(* Logix 5000 AddOnInstructionDefinition export Banner_DXMR_IOLM_Param_v5; software revision 33.00 *)

TYPE Banner_IOL_Port_v5 :   // UDT that has all of the data items necessary to communicate with a specific Port on a IO-Link Master
STRUCT
   Port_Controlled : INT;   // Each bit represents a port on an IO-Link Master. Set to 1 to tell AOI to control that port.
   Port_Activate : INT;   // Each bit represents a port on an IO-Link Master. When ON that port will process any commands in queue.
   Port_Read : INT;   // Each bit represents a port on an IO-Link Master. Used to determine when device AOI has requested a Read command.
   Port_Write : INT;   // Each bit represents a port on an IO-Link Master. Used to determine when device AOI has requested a Write command.
   Port_RW_Complete : INT;   // Each bit represents a port on an IO-Link Master. Tells device AOI that Read or Write request has been completed.
   Port_Device_Read : INT;
   Data_Transfer : SINT[250];   // Array to transfer data from IO-Master to device AOIs.
END_STRUCT
END_TYPE

TYPE Banner_IOLM_EL_v5 :   // Error Log for Messages to IOLM.
STRUCT
   RW : SINT;   // 0 = Read, 1 = Write.
   Port : SINT;   // Port number that generated error.
   Index : INT;   // IO-Link Index for generated error.
END_STRUCT
END_TYPE

TYPE Banner_IOLM_v5 :   // UDT to control IO-Link Masters.
STRUCT
   Message_Source_Data : SINT[260];
   Message_Destination_Data : SINT[260];
   Error_Log : Banner_IOLM_EL_v5[10];
   Error_Write_Retry : BOOL;
   Num_Error_MSGS : DINT;
   IO_Link_Master_Busy : BOOL;   // 0 = While waiting for a command, 1 = Processing command
   AOI_Reset : BOOL;
   Port_Data : Banner_IOL_Port_v5;   // All of the necessary data to work with the various ports of the IO-Link Master.
   Halt_Operation : BOOL;   // When parameter is 1 the AOI is halted as next available time frame.
   AOI_Halted : BOOL;   // AOI is in standby mode until Halt Operation tag is set back to 0.
END_STRUCT
END_TYPE

ADD_ON_INSTRUCTION Banner_DXMR_IOLM_Param_v5   (* revision 5.0, vendor Banner Engineering *)
// AOI that controls a Banner IO-Link Master with IO-Link Devices
// Revision note:
// Added Port Control functionality. This should simplify the setup. Also added links for direct connection to the Input and Output Assmebly Instances.
VAR_IN_OUT
   IOLM : Banner_IOLM_v5; {required}
   Input : SINT[456]; {required}
   Output : SINT[456]; {required}
END_VAR
VAR_INPUT
   Port1 : BOOL; {required}
   Port2 : BOOL; {required}
   Port3 : BOOL; {required}
   Port4 : BOOL; {required}
   Port5 : BOOL; {required}
   Port6 : BOOL; {required}
   Port7 : BOOL; {required}
   Port8 : BOOL; {required}
END_VAR
VAR_OUTPUT
   Done : BOOL; {visible}
   Busy : BOOL; {visible}
   Error : BOOL; {visible}
END_VAR
VAR
   Lock : DINT; {access None}
   Byte_Length : SINT; {access None}
   Current_Port : INT; {access None}   // Current port to communicate with via the IO-Link Master.
   Timer : TIMER := (PRE := 500); {access None}
   Error_Index : DINT; {access None}
   Timer2 : TIMER := (PRE := 5000); {access None}
   Temp_Index : INT; {access None}
   ErrCount : DINT; {access None}
   Timer4 : TIMER := (PRE := 2000); {access None}
   Timer5 : TIMER := (PRE := 2000); {access None}
   Timer3 : TIMER := (PRE := 2000); {access None}
   Timer6 : TIMER := (PRE := 3000); {access None}
   Timer7 : TIMER := (PRE := 3000); {access None}
   Timer8 : TIMER := (PRE := 3000); {access None}
   Write_Index : DINT; {access None}
   WriteTimer : TIMER := (PRE := 60000); {access None}
   WriteCnt : DINT; {access None}
   Last_Index : DINT; {access None}
   WrCntTotal : DINT; {access None}
END_VAR

ROUTINE Logic   (* ladder *)
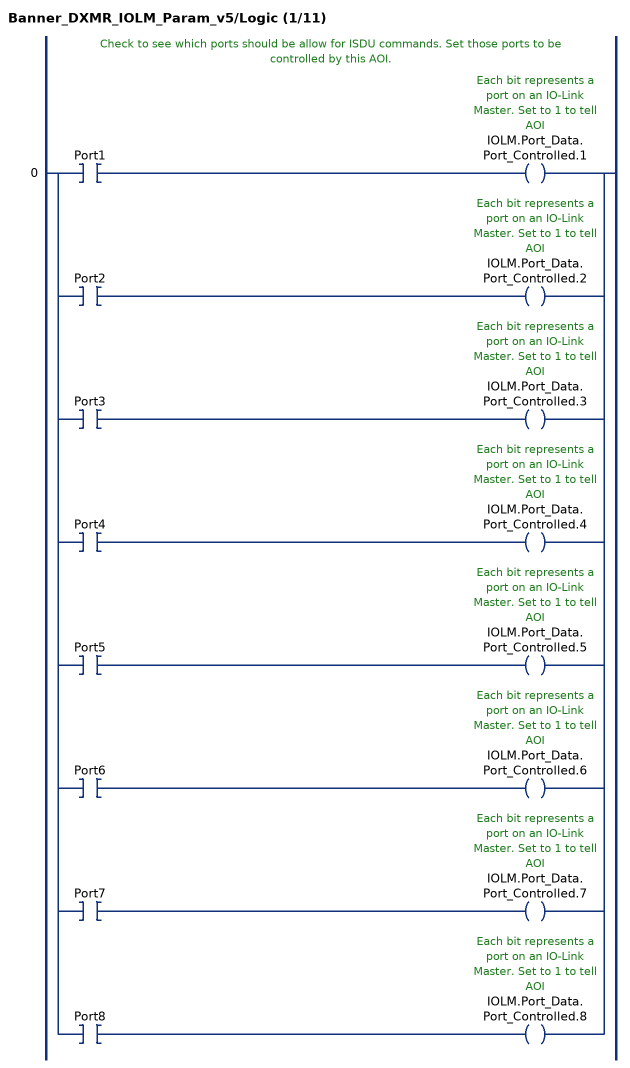
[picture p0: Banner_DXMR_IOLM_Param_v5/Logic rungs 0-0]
   // Check to see which ports should be allow for ISDU commands. Set those ports to be controlled by this AOI.
   0: [XIC(Port1) OTE(IOLM.Port_Data.Port_Controlled.1) ,XIC(Port2) OTE(IOLM.Port_Data.Port_Controlled.2) ,XIC(Port3) OTE(IOLM.Port_Data.Port_Controlled.3) ,XIC(Port4) OTE(IOLM.Port_Data.Port_Controlled.4) ,XIC(Port5) OTE(IOLM.Port_Data.Port_Controlled.5) ,XIC(Port6) OTE(IOLM.Port_Data.Port_Controlled.6) ,XIC(Port7) OTE(IOLM.Port_Data.Port_Controlled.7) ,XIC(Port8) OTE(IOLM.Port_Data.Port_Controlled.8) ];
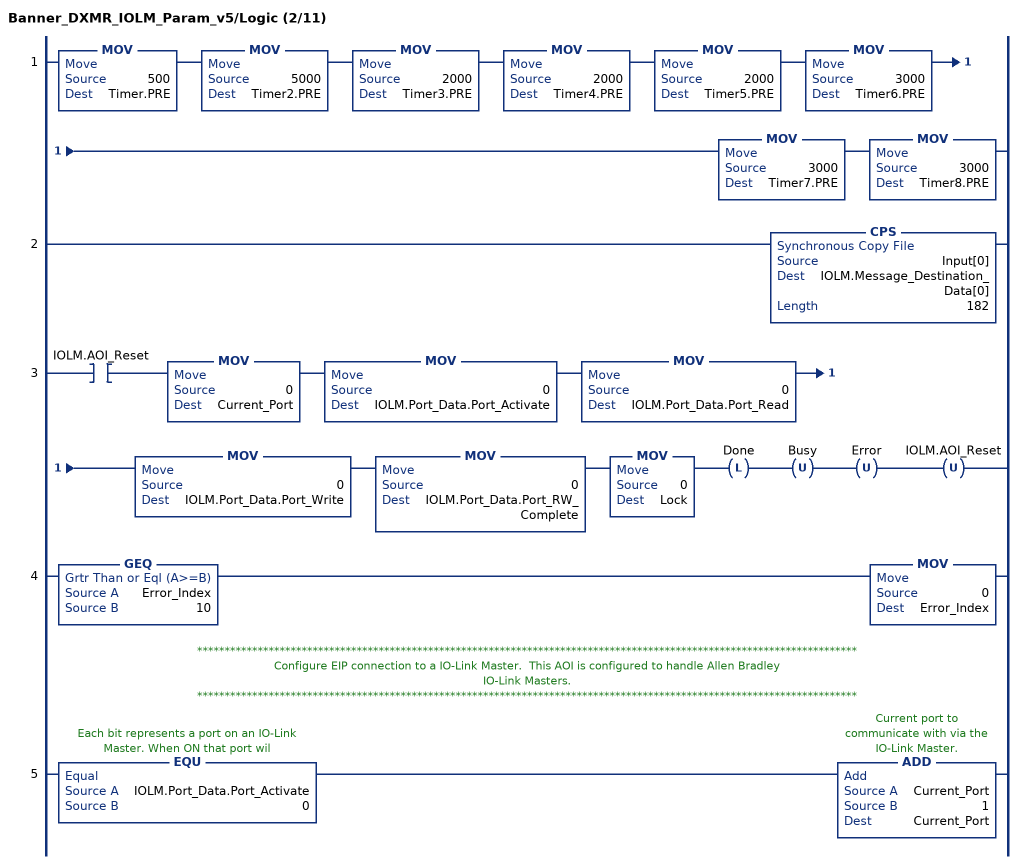
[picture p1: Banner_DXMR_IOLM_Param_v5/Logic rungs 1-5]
   1: MOV(500,Timer.PRE)MOV(5000,Timer2.PRE)MOV(2000,Timer3.PRE)MOV(2000,Timer4.PRE)MOV(2000,Timer5.PRE)MOV(3000,Timer6.PRE)MOV(3000,Timer7.PRE)MOV(3000,Timer8.PRE);
   2: CPS(Input[0],IOLM.Message_Destination_Data[0],182);
   3: XIC(IOLM.AOI_Reset)MOV(0,Current_Port)MOV(0,IOLM.Port_Data.Port_Activate)MOV(0,IOLM.Port_Data.Port_Read)MOV(0,IOLM.Port_Data.Port_Write)MOV(0,IOLM.Port_Data.Port_RW_Complete)MOV(0,Lock)OTL(Done)OTU(Busy)OTU(Error)OTU(IOLM.AOI_Reset);
   4: GEQ(Error_Index,10)MOV(0,Error_Index);
   // ************************************************************************************************************************
   // Configure EIP connection to a IO-Link Master.  This AOI is configured to handle Allen Bradley
   // IO-Link Masters.
   // ************************************************************************************************************************
   5: EQU(IOLM.Port_Data.Port_Activate,0)ADD(Current_Port,1,Current_Port);
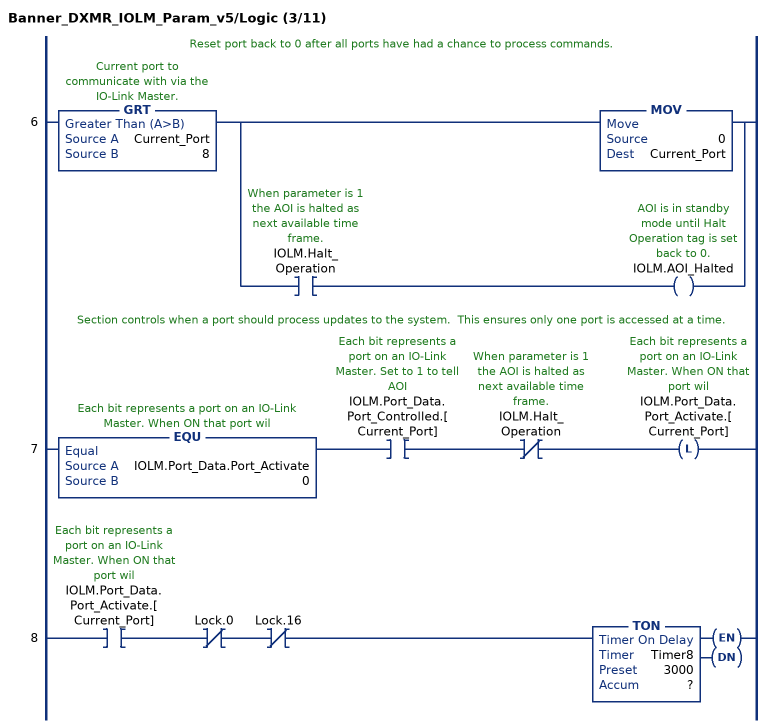
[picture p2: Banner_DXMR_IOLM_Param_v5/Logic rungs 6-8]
   // Reset port back to 0 after all ports have had a chance to process commands.
   6: GRT(Current_Port,8)[MOV(0,Current_Port) ,XIC(IOLM.Halt_Operation) OTE(IOLM.AOI_Halted) ];
   // Section controls when a port should process updates to the system.  This ensures only one port is accessed at a time.
   7: EQU(IOLM.Port_Data.Port_Activate,0)XIC(IOLM.Port_Data.Port_Controlled.[Current_Port])XIO(IOLM.Halt_Operation)OTL(IOLM.Port_Data.Port_Activate.[Current_Port]);
   8: XIC(IOLM.Port_Data.Port_Activate.[Current_Port])XIO(Lock.0)XIO(Lock.16)TON(Timer8,?,?);
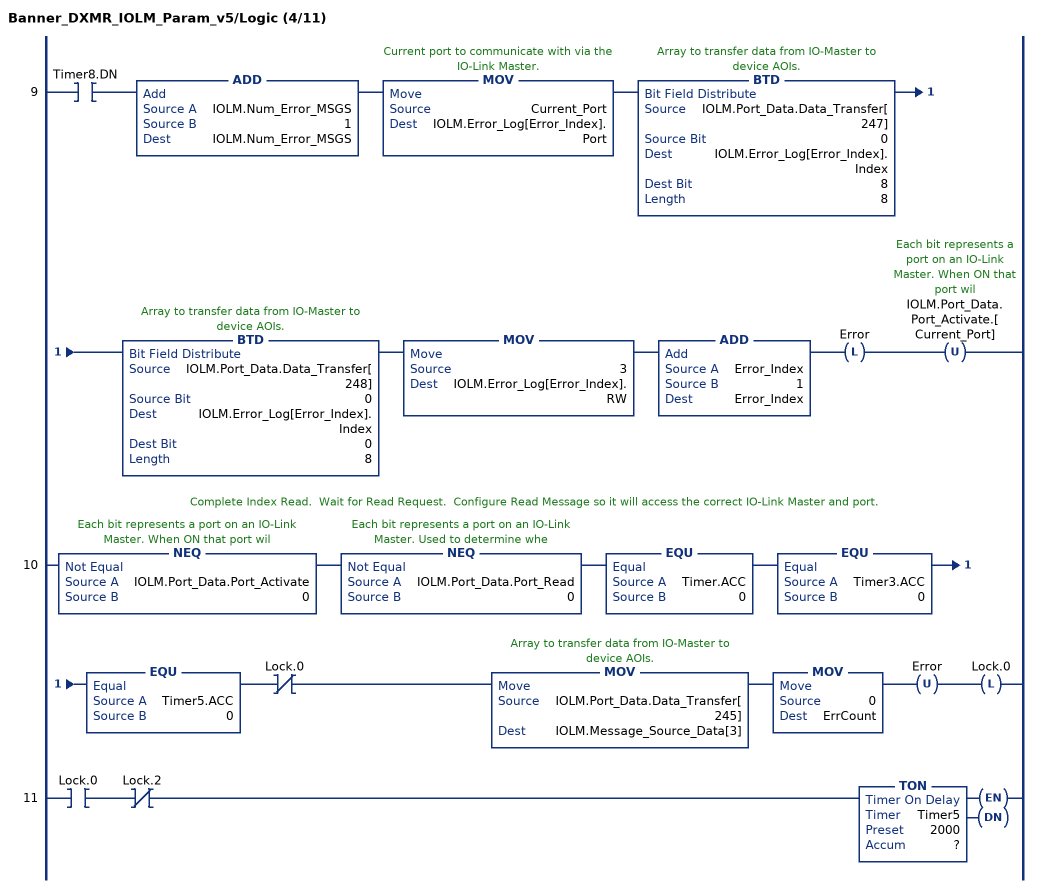
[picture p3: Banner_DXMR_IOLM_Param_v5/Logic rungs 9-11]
   9: XIC(Timer8.DN)ADD(IOLM.Num_Error_MSGS,1,IOLM.Num_Error_MSGS)MOV(Current_Port,IOLM.Error_Log[Error_Index].Port)BTD(IOLM.Port_Data.Data_Transfer[247],0,IOLM.Error_Log[Error_Index].Index,8,8)BTD(IOLM.Port_Data.Data_Transfer[248],0,IOLM.Error_Log[Error_Index].Index,0,8)MOV(3,IOLM.Error_Log[Error_Index].RW)ADD(Error_Index,1,Error_Index)OTL(Error)OTU(IOLM.Port_Data.Port_Activate.[Current_Port]);
   // Complete Index Read.  Wait for Read Request.  Configure Read Message so it will access the correct IO-Link Master and port.
   10: NEQ(IOLM.Port_Data.Port_Activate,0)NEQ(IOLM.Port_Data.Port_Read,0)EQU(Timer.ACC,0)EQU(Timer3.ACC,0)EQU(Timer5.ACC,0)XIO(Lock.0)MOV(IOLM.Port_Data.Data_Transfer[245],IOLM.Message_Source_Data[3])MOV(0,ErrCount)OTU(Error)OTL(Lock.0);
   11: XIC(Lock.0)XIO(Lock.2)TON(Timer5,?,?);
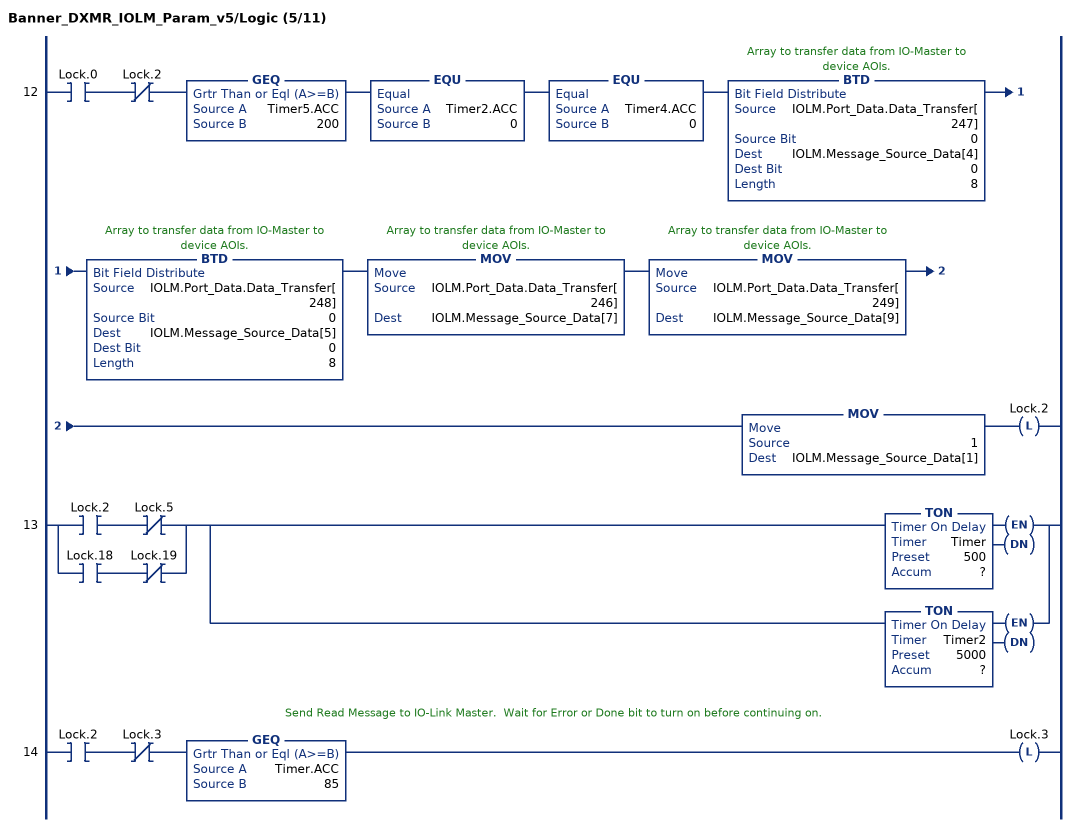
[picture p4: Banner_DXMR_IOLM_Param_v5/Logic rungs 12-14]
   12: XIC(Lock.0)XIO(Lock.2)GEQ(Timer5.ACC,200)EQU(Timer2.ACC,0)EQU(Timer4.ACC,0)BTD(IOLM.Port_Data.Data_Transfer[247],0,IOLM.Message_Source_Data[4],0,8)BTD(IOLM.Port_Data.Data_Transfer[248],0,IOLM.Message_Source_Data[5],0,8)MOV(IOLM.Port_Data.Data_Transfer[246],IOLM.Message_Source_Data[7])MOV(IOLM.Port_Data.Data_Transfer[249],IOLM.Message_Source_Data[9])MOV(1,IOLM.Message_Source_Data[1])OTL(Lock.2);
   13: [XIC(Lock.2) XIO(Lock.5) ,XIC(Lock.18) XIO(Lock.19) ][TON(Timer,?,?) ,TON(Timer2,?,?) ];
   // Send Read Message to IO-Link Master.  Wait for Error or Done bit to turn on before continuing on.
   14: XIC(Lock.2)XIO(Lock.3)GEQ(Timer.ACC,85)OTL(Lock.3);
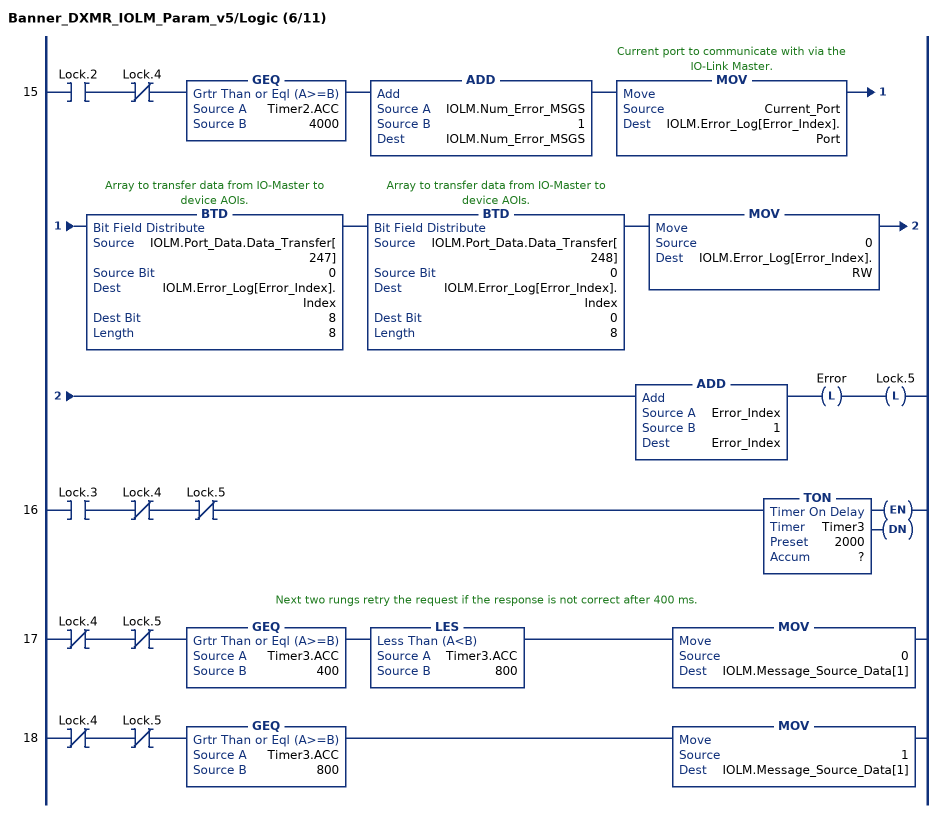
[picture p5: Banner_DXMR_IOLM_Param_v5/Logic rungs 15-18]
   15: XIC(Lock.2)XIO(Lock.4)GEQ(Timer2.ACC,4000)ADD(IOLM.Num_Error_MSGS,1,IOLM.Num_Error_MSGS)MOV(Current_Port,IOLM.Error_Log[Error_Index].Port)BTD(IOLM.Port_Data.Data_Transfer[247],0,IOLM.Error_Log[Error_Index].Index,8,8)BTD(IOLM.Port_Data.Data_Transfer[248],0,IOLM.Error_Log[Error_Index].Index,0,8)MOV(0,IOLM.Error_Log[Error_Index].RW)ADD(Error_Index,1,Error_Index)OTL(Error)OTL(Lock.5);
   16: XIC(Lock.3)XIO(Lock.4)XIO(Lock.5)TON(Timer3,?,?);
   // Next two rungs retry the request if the response is not correct after 400 ms.
   17: XIO(Lock.4)XIO(Lock.5)GEQ(Timer3.ACC,400)LES(Timer3.ACC,800)MOV(0,IOLM.Message_Source_Data[1]);
   18: XIO(Lock.4)XIO(Lock.5)GEQ(Timer3.ACC,800)MOV(1,IOLM.Message_Source_Data[1]);
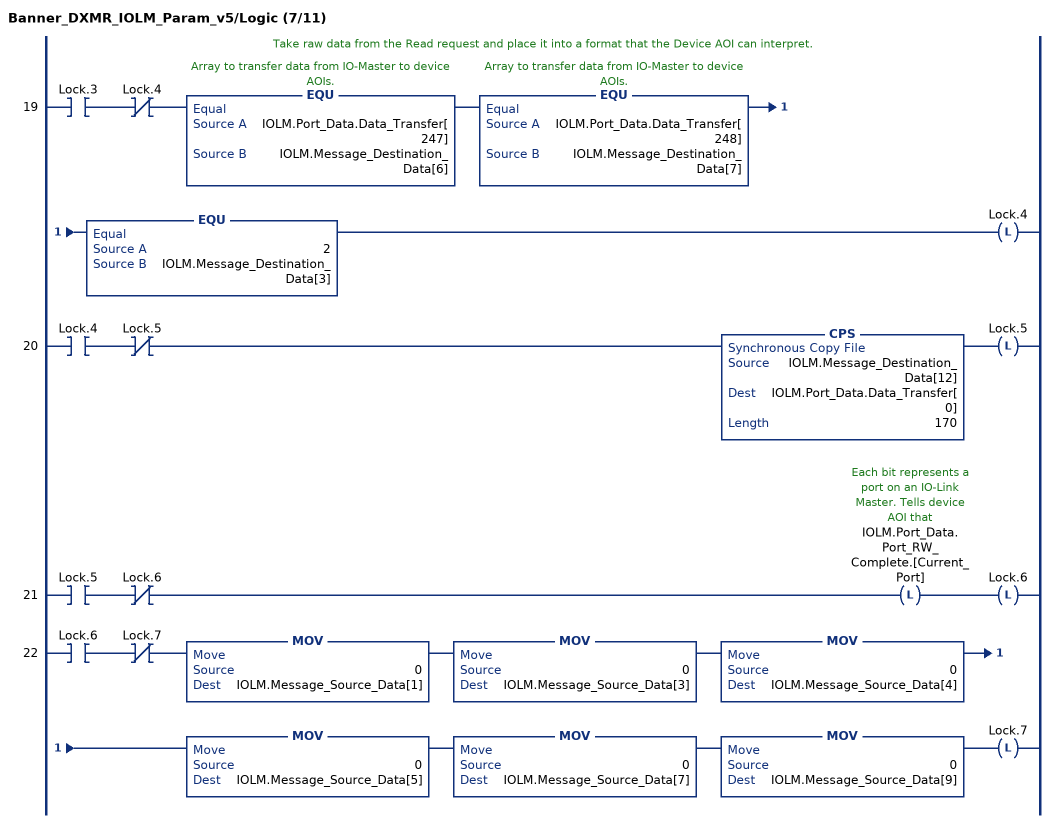
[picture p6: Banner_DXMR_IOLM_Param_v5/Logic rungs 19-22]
   // Take raw data from the Read request and place it into a format that the Device AOI can interpret.
   19: XIC(Lock.3)XIO(Lock.4)EQU(IOLM.Port_Data.Data_Transfer[247],IOLM.Message_Destination_Data[6])EQU(IOLM.Port_Data.Data_Transfer[248],IOLM.Message_Destination_Data[7])EQU(2,IOLM.Message_Destination_Data[3])OTL(Lock.4);
   20: XIC(Lock.4)XIO(Lock.5)CPS(IOLM.Message_Destination_Data[12],IOLM.Port_Data.Data_Transfer[0],170)OTL(Lock.5);
   21: XIC(Lock.5)XIO(Lock.6)OTL(IOLM.Port_Data.Port_RW_Complete.[Current_Port])OTL(Lock.6);
   22: XIC(Lock.6)XIO(Lock.7)MOV(0,IOLM.Message_Source_Data[1])MOV(0,IOLM.Message_Source_Data[3])MOV(0,IOLM.Message_Source_Data[4])MOV(0,IOLM.Message_Source_Data[5])MOV(0,IOLM.Message_Source_Data[7])MOV(0,IOLM.Message_Source_Data[9])OTL(Lock.7);
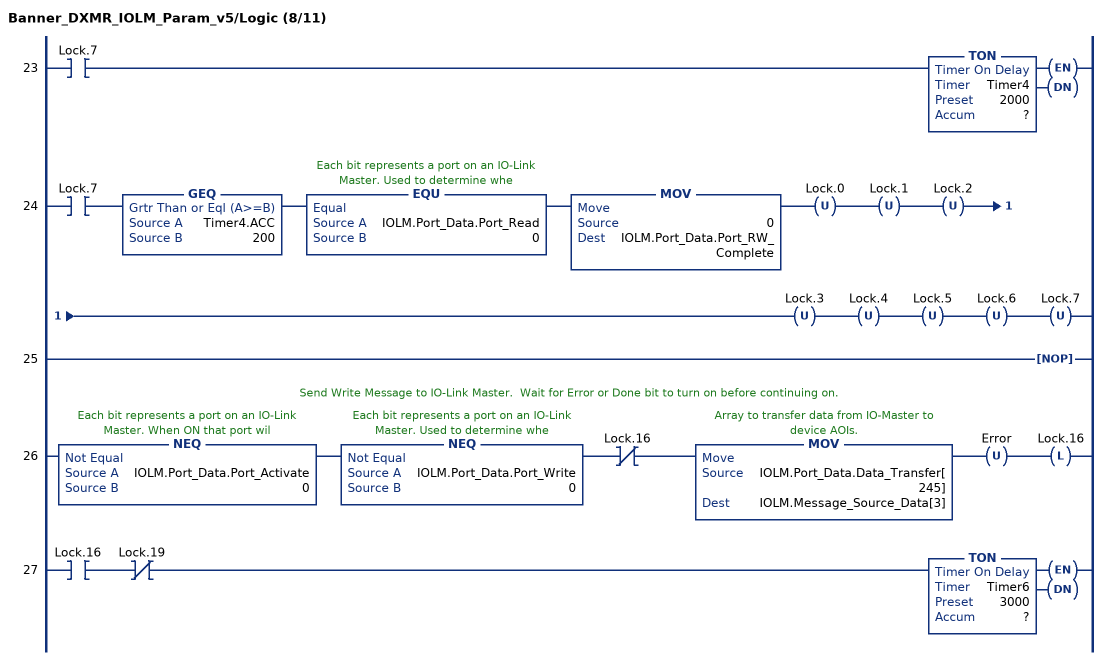
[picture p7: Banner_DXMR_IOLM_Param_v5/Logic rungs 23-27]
   23: XIC(Lock.7)TON(Timer4,?,?);
   24: XIC(Lock.7)GEQ(Timer4.ACC,200)EQU(IOLM.Port_Data.Port_Read,0)MOV(0,IOLM.Port_Data.Port_RW_Complete)OTU(Lock.0)OTU(Lock.1)OTU(Lock.2)OTU(Lock.3)OTU(Lock.4)OTU(Lock.5)OTU(Lock.6)OTU(Lock.7);
   25: NOP();
   // Send Write Message to IO-Link Master.  Wait for Error or Done bit to turn on before continuing on.
   26: NEQ(IOLM.Port_Data.Port_Activate,0)NEQ(IOLM.Port_Data.Port_Write,0)XIO(Lock.16)MOV(IOLM.Port_Data.Data_Transfer[245],IOLM.Message_Source_Data[3])OTU(Error)OTL(Lock.16);
   27: XIC(Lock.16)XIO(Lock.19)TON(Timer6,?,?);
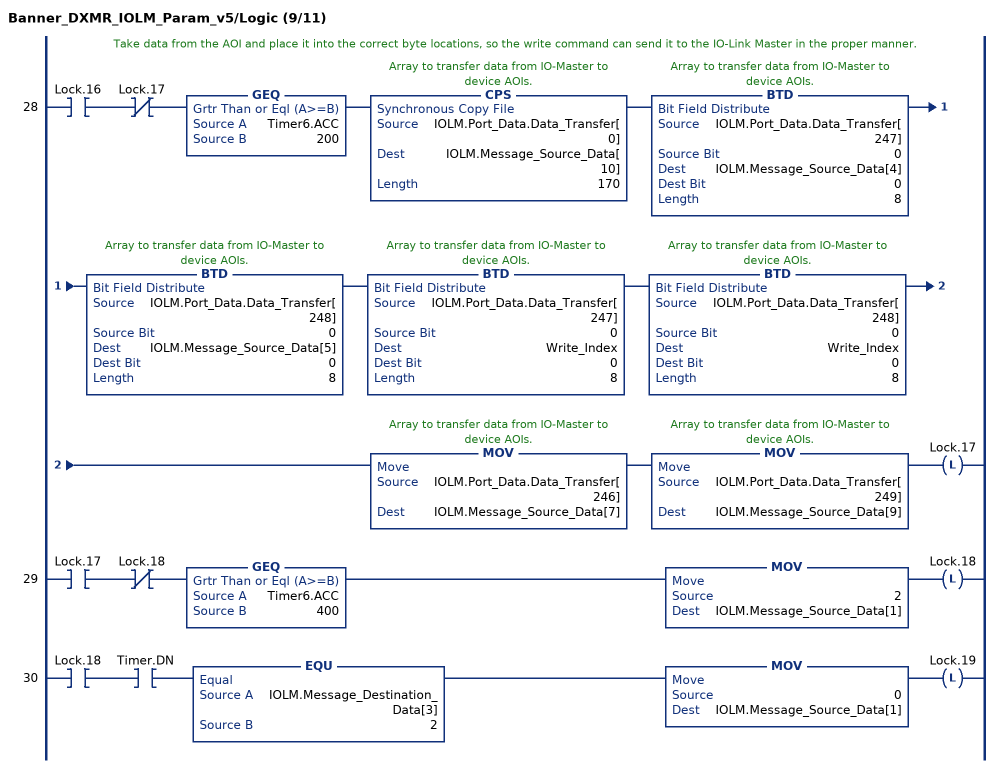
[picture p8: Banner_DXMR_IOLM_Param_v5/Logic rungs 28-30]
   // Take data from the AOI and place it into the correct byte locations, so the write command can send it to the IO-Link Master in the proper manner.
   28: XIC(Lock.16)XIO(Lock.17)GEQ(Timer6.ACC,200)CPS(IOLM.Port_Data.Data_Transfer[0],IOLM.Message_Source_Data[10],170)BTD(IOLM.Port_Data.Data_Transfer[247],0,IOLM.Message_Source_Data[4],0,8)BTD(IOLM.Port_Data.Data_Transfer[248],0,IOLM.Message_Source_Data[5],0,8)BTD(IOLM.Port_Data.Data_Transfer[247],0,Write_Index,0,8)BTD(IOLM.Port_Data.Data_Transfer[248],0,Write_Index,0,8)MOV(IOLM.Port_Data.Data_Transfer[246],IOLM.Message_Source_Data[7])MOV(IOLM.Port_Data.Data_Transfer[249],IOLM.Message_Source_Data[9])OTL(Lock.17);
   29: XIC(Lock.17)XIO(Lock.18)GEQ(Timer6.ACC,400)MOV(2,IOLM.Message_Source_Data[1])OTL(Lock.18);
   30: XIC(Lock.18)XIC(Timer.DN)EQU(IOLM.Message_Destination_Data[3],2)MOV(0,IOLM.Message_Source_Data[1])OTL(Lock.19);
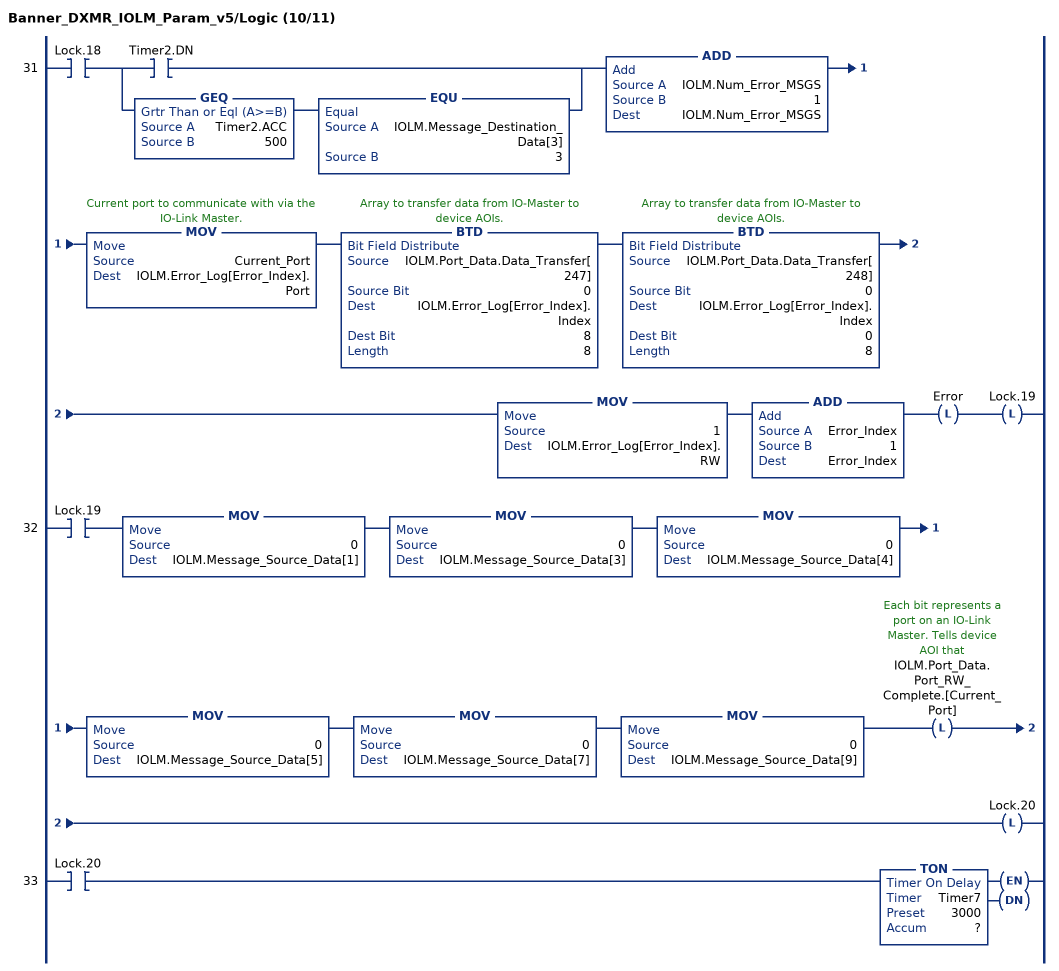
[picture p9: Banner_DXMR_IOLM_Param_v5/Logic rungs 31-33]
   31: XIC(Lock.18)[XIC(Timer2.DN) ,GEQ(Timer2.ACC,500) EQU(IOLM.Message_Destination_Data[3],3) ]ADD(IOLM.Num_Error_MSGS,1,IOLM.Num_Error_MSGS)MOV(Current_Port,IOLM.Error_Log[Error_Index].Port)BTD(IOLM.Port_Data.Data_Transfer[247],0,IOLM.Error_Log[Error_Index].Index,8,8)BTD(IOLM.Port_Data.Data_Transfer[248],0,IOLM.Error_Log[Error_Index].Index,0,8)MOV(1,IOLM.Error_Log[Error_Index].RW)ADD(Error_Index,1,Error_Index)OTL(Error)OTL(Lock.19);
   32: XIC(Lock.19)MOV(0,IOLM.Message_Source_Data[1])MOV(0,IOLM.Message_Source_Data[3])MOV(0,IOLM.Message_Source_Data[4])MOV(0,IOLM.Message_Source_Data[5])MOV(0,IOLM.Message_Source_Data[7])MOV(0,IOLM.Message_Source_Data[9])OTL(IOLM.Port_Data.Port_RW_Complete.[Current_Port])OTL(Lock.20);
   33: XIC(Lock.20)TON(Timer7,?,?);
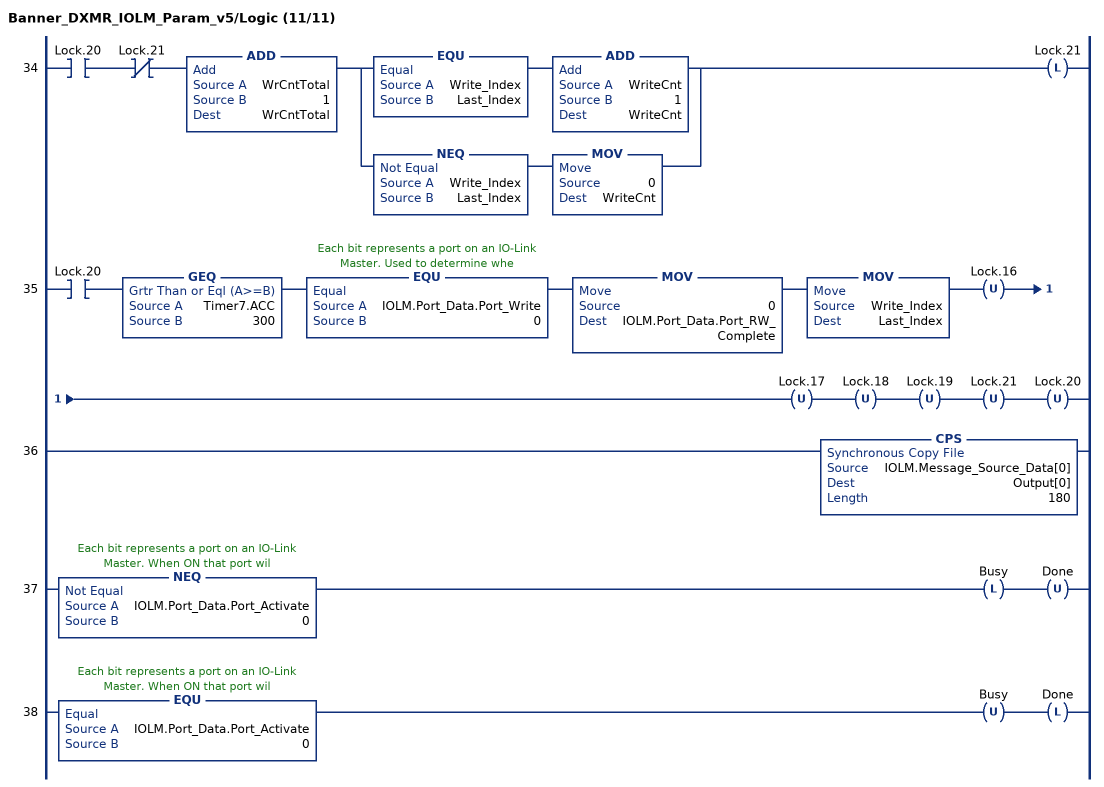
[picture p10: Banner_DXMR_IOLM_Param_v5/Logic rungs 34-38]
   34: XIC(Lock.20)XIO(Lock.21)ADD(WrCntTotal,1,WrCntTotal)[EQU(Write_Index,Last_Index) ADD(WriteCnt,1,WriteCnt) ,NEQ(Write_Index,Last_Index) MOV(0,WriteCnt) ]OTL(Lock.21);
   35: XIC(Lock.20)GEQ(Timer7.ACC,300)EQU(IOLM.Port_Data.Port_Write,0)MOV(0,IOLM.Port_Data.Port_RW_Complete)MOV(Write_Index,Last_Index)OTU(Lock.16)OTU(Lock.17)OTU(Lock.18)OTU(Lock.19)OTU(Lock.21)OTU(Lock.20);
   36: CPS(IOLM.Message_Source_Data[0],Output[0],180);
   37: NEQ(IOLM.Port_Data.Port_Activate,0)OTL(Busy)OTU(Done);
   38: EQU(IOLM.Port_Data.Port_Activate,0)OTU(Busy)OTL(Done);
END_ROUTINE
END_ADD_ON_INSTRUCTION
